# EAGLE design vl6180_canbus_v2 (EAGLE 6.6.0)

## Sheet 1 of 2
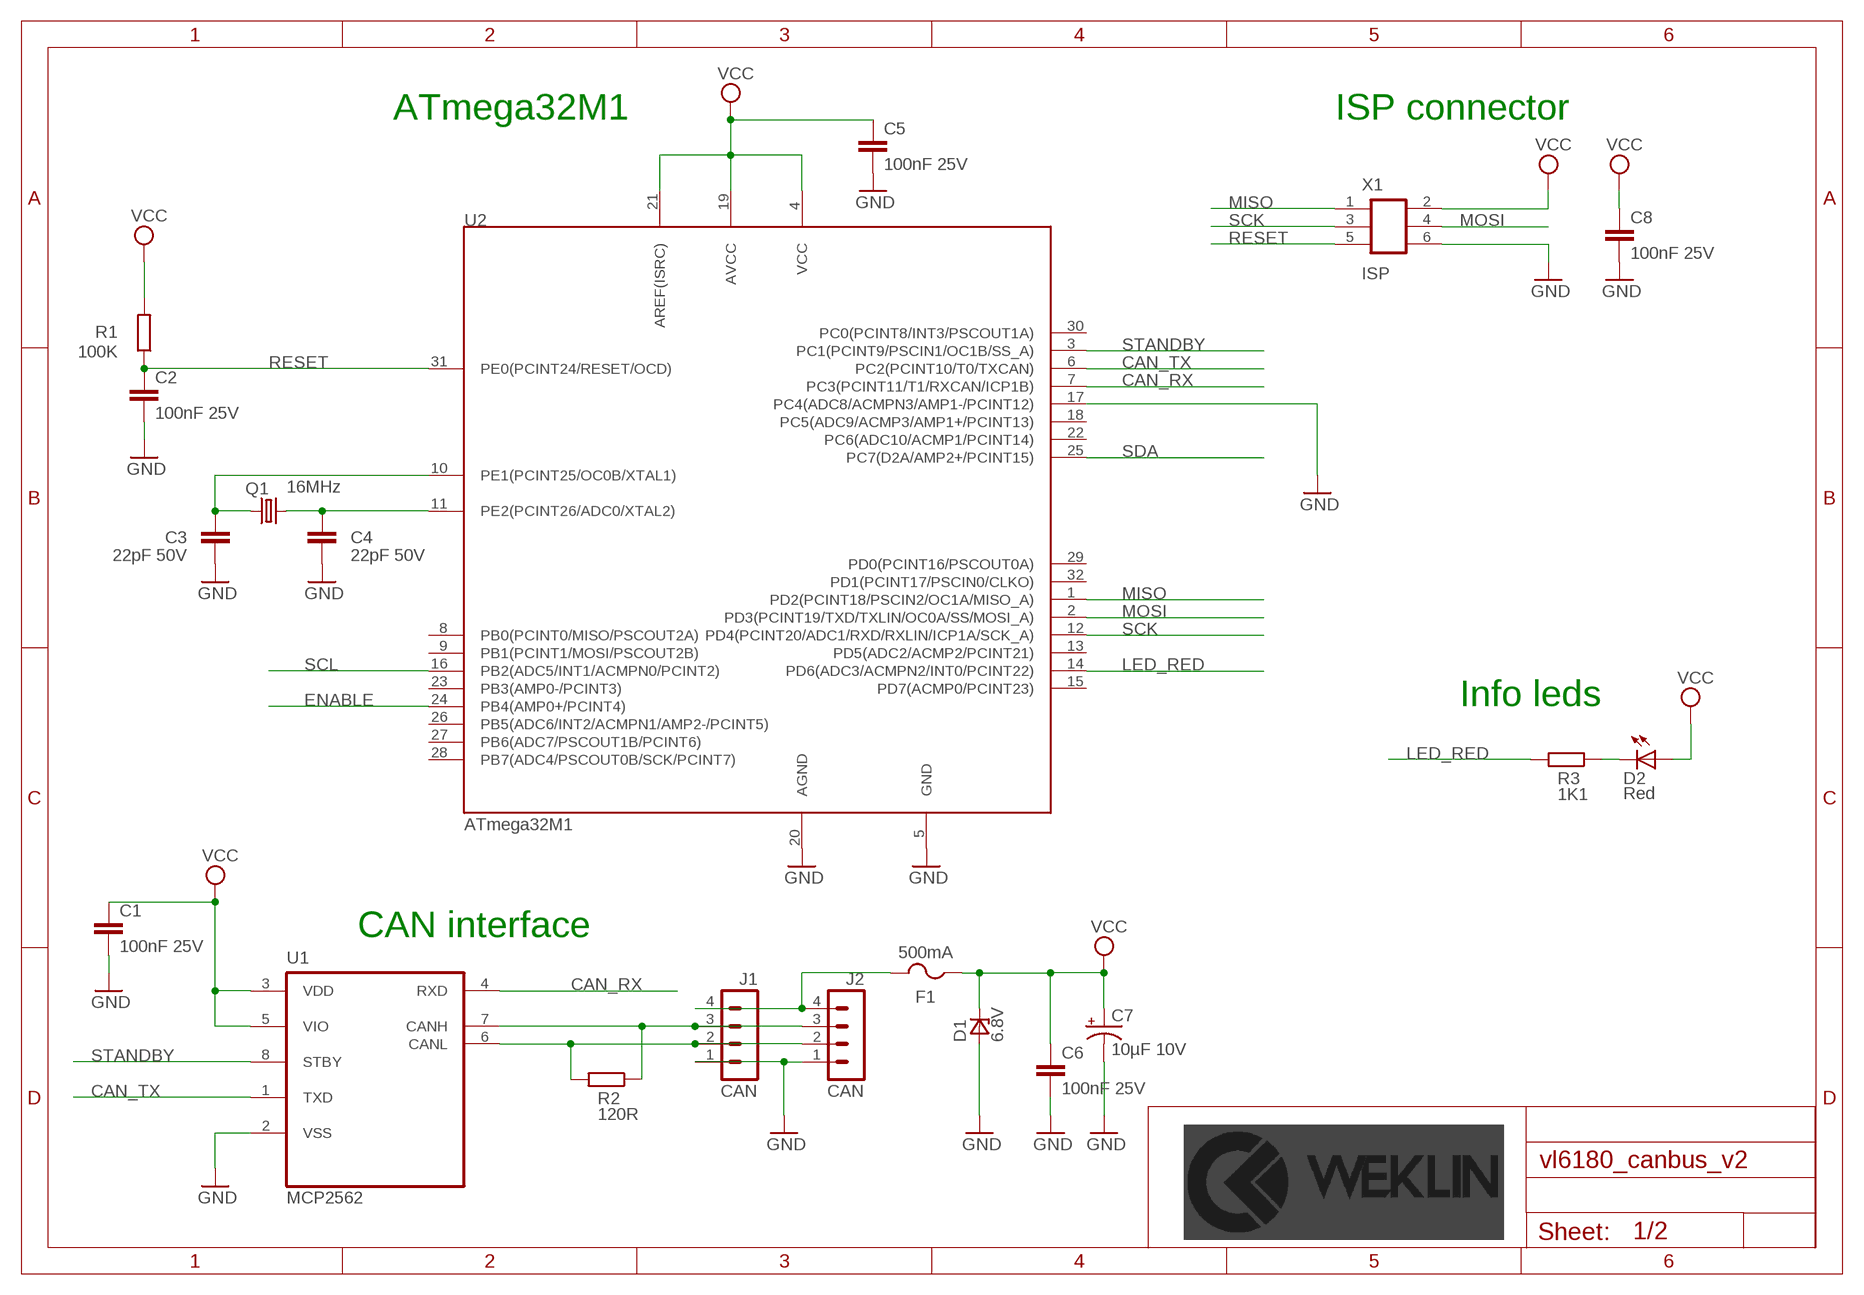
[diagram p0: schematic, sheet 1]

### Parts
C1  100nF 25V  CAPACITOR_NON_POL-100NF-25V(+-10%)(2012)  [C2012]
C2  100nF 25V  CAPACITOR_NON_POL-100NF-25V(+-10%)(2012)  [C2012]
C3  22pF 50V  CAPACITOR_NON_POL-22PF-50V(+-5%)(2012)  [C2012]
C4  22pF 50V  CAPACITOR_NON_POL-22PF-50V(+-5%)(2012)  [C2012]
C5  100nF 25V  CAPACITOR_NON_POL-100NF-25V(+-10%)(2012)  [C2012]
C6  100nF 25V  CAPACITOR_NON_POL-100NF-25V(+-10%)(2012)  [C2012]
C7  10µF 10V  CAPACITOR_POL-10µF-10V(+-10%)(3216)  [EIA3216]
C8  100nF 25V  CAPACITOR_NON_POL-100NF-25V(+-10%)(2012)  [C2012]
D1  6.8V  ZENER_UNIDIR6.8  [DO-214AA]
D2  Red  LEDVLDS1235G  [VLD]
F1  500mA  FUSE0451.500MRL  [EIARS-481-2]
J1  CAN  MICROLOCK-4CMS_VERTICAL  [504194-0470]
J2  CAN  MICROLOCK-4CMS_VERTICAL  [504194-0470]
Q1  16MHz  CRYSTAL-16MHZ_SMD(3225)  [SMD_KX7]
R1  100K  RESISTOR-100K(+-1%)(2012)  [R2012]
R2  120R  RESISTOR-120R(+-1%)(2012)  [R2012]
R3  1K1  RESISTOR-1K1(+-1%)(2012)  [R2012]
U1  MCP2562  MCP2562-E/SN-SOIC8  [SOIC8]
U2  ATmega32M1  ATMEGA32M1-TQFP32  [TQFP32]
X1  ISP  CON_2X3-SMD_1.27MM_MALE  [2X3_1.27MM_MALE_SMD]

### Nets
CAN_RX: U1.4(RXD) U2.7(PC3(PCINT11/T1/RXCAN/ICP1B))
CAN_TX: U1.1(TXD) U2.6(PC2(PCINT10/T0/TXCAN))
ENABLE: U2.24(PB4(AMP0+/PCINT4)) ; also sheet 2
GND: C1.2 C2.2 C3.2 C4.2 C5.2 C6.2 C7.C(-) C8.2 D1.A J1.1 J2.1 U1.2(VSS) U2.5(GND) U2.17(PC4(ADC8/ACMPN3/AMP1-/PCINT12)) U2.20(AGND) X1.6 ; also sheet 2
LED_RED: R3.2 U2.14(PD6(ADC3/ACMPN2/INT0/PCINT22))
MISO: U2.1(PD2(PCINT18/PSCIN2/OC1A/MISO_A)) X1.1
MOSI: U2.2(PD3(PCINT19/TXD/TXLIN/OC0A/SS/MOSI_A)) X1.4
N$2: D2.C R3.1
N$4: F1.2 J1.4 J2.4
N$5: J1.2 J2.2 R2.2 U1.6(CANL)
N$6: J1.3 J2.3 R2.1 U1.7(CANH)
N$7: C4.1 Q1.3 U2.11(PE2(PCINT26/ADC0/XTAL2))
N$9: C3.1 Q1.1 U2.10(PE1(PCINT25/OC0B/XTAL1))
RESET: C2.1 R1.1 U2.31(PE0(PCINT24/RESET/OCD)) X1.5
SCK: U2.12(PD4(PCINT20/ADC1/RXD/RXLIN/ICP1A/SCK_A)) X1.3
SCL: U2.16(PB2(ADC5/INT1/ACMPN0/PCINT2)) ; also sheet 2
SDA: U2.25(PC7(D2A/AMP2+/PCINT15)) ; also sheet 2
STANDBY: U1.8(STBY) U2.3(PC1(PCINT9/PSCIN1/OC1B/SS_A))
VCC: C1.1 C5.1 C6.1 C7.A(+) C8.1 D1.C D2.A F1.1 R1.2 U1.3(VDD) U1.5(VIO) U2.4(VCC) U2.19(AVCC) U2.21(AREF(ISRC)) X1.2 ; also sheet 2
Unconnected: U2.8(PB0(PCINT0/MISO/PSCOUT2A)) U2.9(PB1(PCINT1/MOSI/PSCOUT2B)) U2.13(PD5(ADC2/ACMP2/PCINT21)) U2.15(PD7(ACMP0/PCINT23)) U2.18(PC5(ADC9/ACMP3/AMP1+/PCINT13)) U2.22(PC6(ADC10/ACMP1/PCINT14)) U2.23(PB3(AMP0-/PCINT3)) U2.26(PB5(ADC6/INT2/ACMPN1/AMP2-/PCINT5)) U2.27(PB6(ADC7/PSCOUT1B/PCINT6)) U2.28(PB7(ADC4/PSCOUT0B/SCK/PCINT7)) U2.29(PD0(PCINT16/PSCOUT0A)) U2.30(PC0(PCINT8/INT3/PSCOUT1A)) U2.32(PD1(PCINT17/PSCIN0/CLKO))

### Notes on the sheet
- ATmega32M1 | ISP connector
- Info leds
- CAN interface

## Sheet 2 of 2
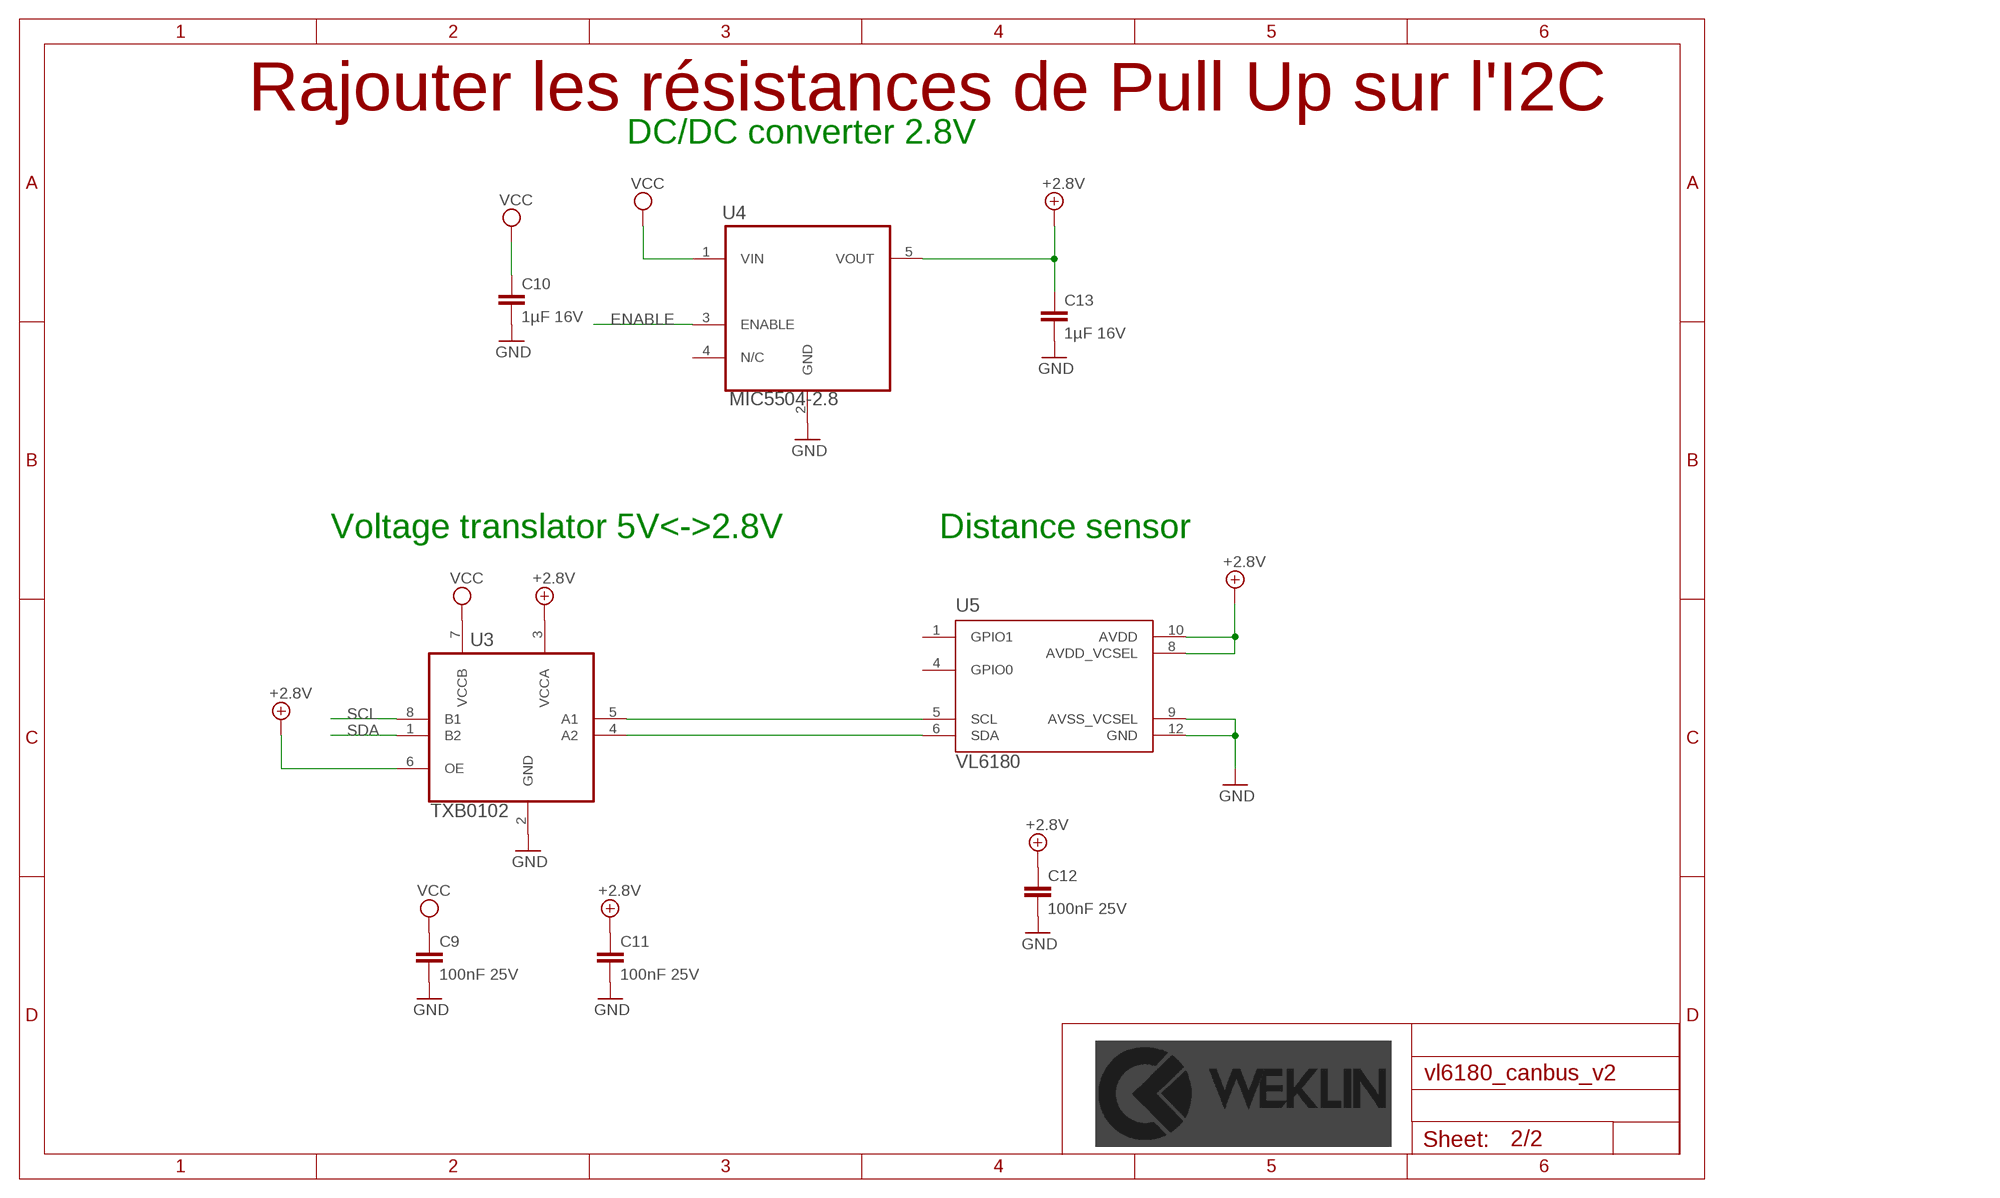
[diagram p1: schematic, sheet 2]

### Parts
C9  100nF 25V  CAPACITOR_NON_POL-100NF-25V(+-10%)(2012)  [C2012]
C10  1µF 16V  CAPACITOR_NON_POL-1µF-16V(-20%)(2012)  [C2012]
C11  100nF 25V  CAPACITOR_NON_POL-100NF-25V(+-10%)(2012)  [C2012]
C12  100nF 25V  CAPACITOR_NON_POL-100NF-25V(+-10%)(2012)  [C2012]
C13  1µF 16V  CAPACITOR_NON_POL-1µF-16V(-20%)(2012)  [C2012]
U3  TXB0102  [VSSOP-8]
U4  MIC5504-2.8  MIC5504-2.8M5-TR  [SOT23-5]
U5  VL6180  [VL6180]

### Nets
+2.8V: C11.1 C12.1 C13.1 U3.3(VCCA) U3.6(OE) U4.5(VOUT) U5.8(AVDD_VCSEL) U5.10(AVDD)
ENABLE: U4.3(ENABLE) ; also sheet 1
GND: C9.2 C10.2 C11.2 C12.2 C13.2 U3.2(GND) U4.2(GND) U5.9(AVSS_VCSEL) U5.12(GND) ; also sheet 1
N$8: U3.5(A1) U5.5(SCL)
N$10: U3.4(A2) U5.6(SDA)
SCL: U3.8(B1) ; also sheet 1
SDA: U3.1(B2) ; also sheet 1
VCC: C9.1 C10.1 U3.7(VCCB) U4.1(VIN) ; also sheet 1
Unconnected: U4.4(N/C) U5.1(GPIO1) U5.4(GPIO0)

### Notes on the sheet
- Rajouter les résistances de Pull Up sur l'I2C
- DC/DC converter 2.8V
- Voltage translator 5V<->2.8V | Distance sensor

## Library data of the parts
C1 C2 C5 C6 C8 C9 C11 C12 = weklin_capacitor:CAPACITOR_NON_POL: Condensateur céramique multicouche; LIB: weklin_capacitor; MANUFACTURER: AVX; MPN: 08053C104KAT2A; OC_FARNELL: 2280951; PRICE: 0,0036
C3 C4 = weklin_capacitor:CAPACITOR_NON_POL: Condensateur céramique multicouche; LIB: weklin_capacitor; MANUFACTURER: Multicomp; MPN: MC0805N220J500CT; OC_FARNELL: 2310684; PRICE: 0,0078
C7 = weklin_capacitor:CAPACITOR_POL: Capacitor; LIB: weklin_capacitor; MANUFACTURER: Kemet; MPN: T491A106K010AT; OC_FARNELL: 2250086; PRICE: 0,0578
C10 C13 = weklin_capacitor:CAPACITOR_NON_POL: Condensateur céramique multicouche; LIB: weklin_capacitor; MANUFACTURER: Walsin; MPN: 0805F105Z160CT; OC_FARNELL: 2495495; PRICE: 0,0097
D1 = weklin_diode:ZENER_UNIDIR: P6SMBxxA Series of unidirectional Transient Voltage Suppressor Diodes; LIB: weklin_diode; MANUFACTURER: ON Semiconductor; MPN: P6SMB6.8AT3G; OC_FARNELL: 1459166RL; PRICE: 0,178
D2 = weklin_led:LED: Led; LIB: weklin_led; MANUFACTURER: Vishay; MPN: VLDS1235G; OC_FARNELL: 2494682; PRICE: 0,003
F1 = weklin_fuse:FUSE: Fuse; LIB: weklin_fuse; MANUFACTURER: Littlefuse; MPN: 0451500MRL; OC_FARNELL: 2383271; PRICE: 0,527
J1 J2 = weklin_micro-lock:MICROLOCK-4: Connecteur MOLEX de 4 Contacts Série Mini50 GEII/IUT ANGERS; LIB: weklin_micro-lock; MANUFACTURER: Molex; MPN: 504194-0470; OC_FARNELL: 2445424; PRICE: 0,232
Q1 = weklin_crystal:CRYSTAL: Crystal resonator; LIB: weklin_crystal; MANUFACTURER: AEL CRYSTALS; MPN: E3SB16.0000F09G11AE; OC_FARNELL: 2467444RL; PRICE: 0,315
R1 = weklin_resistor:RESISTOR: Resistor; LIB: weklin_resistor; MANUFACTURER: Multicomp; MPN: MCWR08X1003FTL; OC_FARNELL: 2446868; PRICE: 0,0014
R2 = weklin_resistor:RESISTOR: Resistor; LIB: weklin_resistor; MANUFACTURER: Multicomp; MPN: MCWR08X1200FTL; OC_FARNELL: 2446878; PRICE: 0,0014
R3 = weklin_resistor:RESISTOR: Resistor; LIB: weklin_resistor; MANUFACTURER: Multicomp; MPN: MC0805S8F1101T5E; OC_FARNELL: 1635316; PRICE: 0,003
U1 = weklin_ic_can:MCP2562-E/SN: High-Speed CAN Transceiver; LIB: weklin_ic_can; MANUFACTURER: Microchip; MPN: MCP2562-E/SN; OC_FARNELL: 2362839; PRICE: 1,12
U2 = weklin_micro-atmell:ATMEGA32M1: ATMEL ATMEGA32M1-AU MCU 8 BITS ATMEGA 16MHZ; LIB: weklin_micro_atmell; MANUFACTURER: Atmel; MPN: ATmega32M1-AU; OC_FARNELL: 2443180; PRICE: 6,18
U3 = weklin_ic_special:TXB0102: Convertisseur de niveau de tension de 1,2V à 5,5V Doc constructeur GEII/IUT ANGERS; LIB: weklin_ic_special; MANUFACTURER: Texas Instrument; MPN: TXB0102DCUR; OC_FARNELL: 2295723; PRICE: 0,962
U4 = weklin_regulator:MIC5504: MICROCHIP MIC5504-2.8YM5-TR Régulateur LDO Tension fixe, 2.5V à 5.5V, 160mV Dropout, 2.8Vout, 300mA, SOT-23-5; LIB: weklin_regulator; MANUFACTURER: Micrel; MNP: MIC5504-2.8YM5-TR; OC_FARNELL: 2510373RL; PRICE: 0.0775
U5 = weklin_sensor:VL6180: Time of flight distance sensor; LIB: weklin_sensor; MANUFACTURER: ST Microelectronics; MPN: VL6180XV0NR/1; OC_FARNELL: 2462820; PRICE: 7,79
X1 = weklin_connector:CON_2X3: Board-To-Board Connector, Micro-MaTch Series, Embase, 6voies.; LIB: weklin_connector; MANUFACTURER: Minitek; MPN: 20021121-00006C4LF; OC_FARNELL: 1865277; PRICE: 0,333

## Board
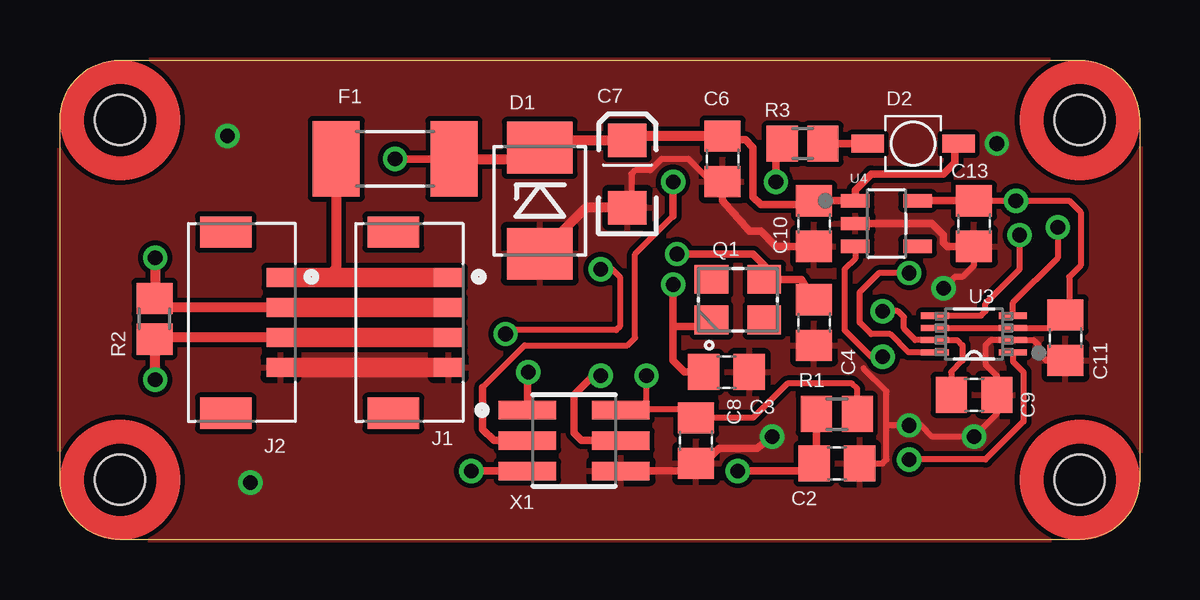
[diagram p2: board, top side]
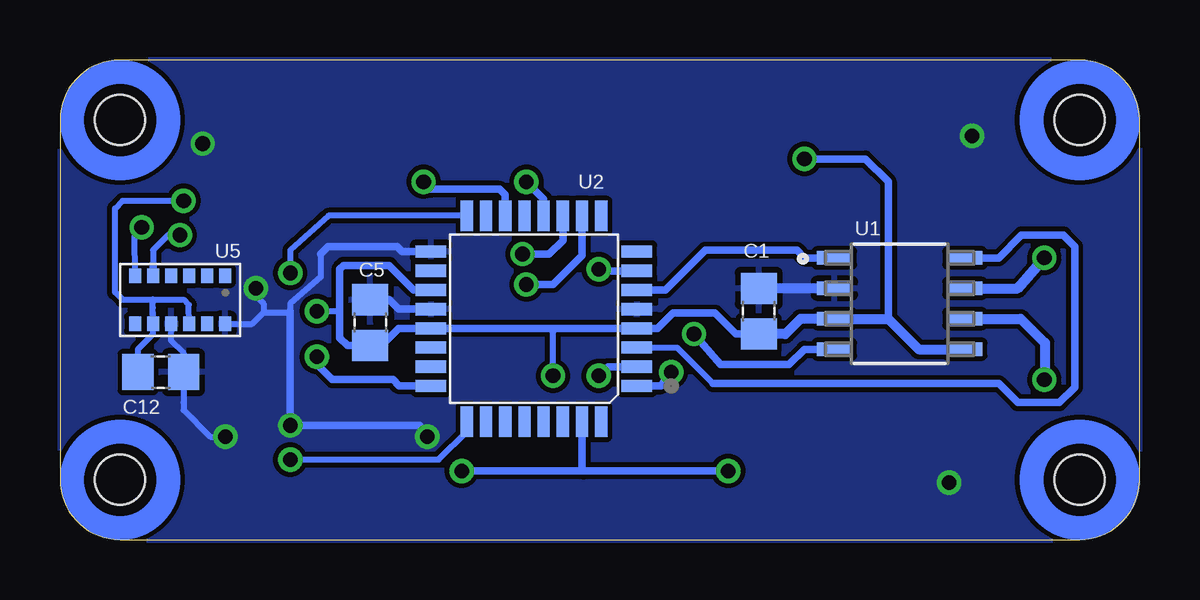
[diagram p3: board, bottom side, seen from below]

Size 45 x 20 mm. Coordinates in mm from the lower left corner, seen from the top.
Outline: 0,2.5 0,17.5 arc-90 2.5,20 42.5,20 arc-90 45,17.5 45,2.5 arc-90 42.5,0 2.5,0 arc-90 0,2.5
Copper layers (1*16): Top 0.035mm / dielectric 1.5mm / Bottom 0.035mm
Design rules "default *": minimum track width 10mil, minimum drill 24mil, track to track 8mil, track to pad 8mil, pad to pad 8mil, via to via 8mil, smd to smd 8mil, copper to edge 0mil, drill to drill 8mil, minimum pad ring 10mil, minimum via ring 8mil, stop-mask expansion 4mil, vias tented up to drill 0mil, thermal gap 10mil
Holes 2.1 mm at 2.5,17.5 42.5,17.5 42.5,2.5 2.5,2.5
tKeepout: area -0.5,14.5 to 5.5,20.5; area -0.5,-0.5 to 5.5,5.5; area 39.5,14.5 to 45.5,20.5; area 39.5,-0.5 to 45.5,5.5; area 2,0 to 42.5,2; area 0,3 to 2,17; area 3,18 to 42.5,20; area 43,3.5 to 45,17
bKeepout: area 3,18 to 42.5,20; area 0,3 to 2,17; area 2,0 to 42.5,2; area 43,3.5 to 45,17; area 39.5,14.5 to 45.5,20.5; area -0.5,14.5 to 5.5,20.5; area -0.5,-0.5 to 5.5,5.5; area 39.5,-0.5 to 45.5,5.5

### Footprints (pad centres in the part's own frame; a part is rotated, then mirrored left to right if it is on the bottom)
C2012 = smd 1.3 x 1.5: 1 -0.95,0; 2 0.95,0
EIA3216 = smd 1.4 x 1.6: A 1.4,0; C -1.4,0
DO-214AA = smd 2.159 x 2.743: A 2.21,0; C -2.21,0
VLD = smd 1.35 x 0.75: A 1.9,0; C -1.9,0
EIARS-481-2 = smd 1.956 x 3.15: 1 -2.451,0; 2 2.451,0
504194-0470 = smd 0.8 x 1.2: 1 -1.875,0; 2 -0.625,0; 3 0.625,0; 4 1.875,0 | smd 1.3 x 2.15: P$5 -3.775,2.295; P$6 3.775,2.295
SMD_KX7 = smd 1.4 x 1.2: 1 -1.1,-0.85; 2 1.1,-0.85; 3 1.1,0.85; 4 -1.1,0.85
R2012 = smd 1.3 x 1.5: 1 -0.85,0; 2 0.85,0
SOIC8 = smd 1.473 x 0.559: 1 -2.718,1.905; 2 -2.718,0.635; 3 -2.718,-0.635; 4 -2.718,-1.905; 5 2.718,-1.905; 6 2.718,-0.635; 7 2.718,0.635; 8 2.718,1.905
TQFP32 = smd 1.27 x 0.508: 1 -4.293,2.8; 2 -4.293,2; 3 -4.293,1.2; 4 -4.293,0.4; 5 -4.293,-0.4; 6 -4.293,-1.2; 7 -4.293,-2; 8 -4.293,-2.8; 17 4.293,-2.8; 18 4.293,-2; 19 4.293,-1.2; 20 4.293,-0.4; 21 4.293,0.4; 22 4.293,1.2; 23 4.293,2; 24 4.293,2.8 | smd 0.508 x 1.27: 9 -2.8,-4.293; 10 -2,-4.293; 11 -1.2,-4.293; 12 -0.4,-4.293; 13 0.4,-4.293; 14 1.2,-4.293; 15 2,-4.293; 16 2.8,-4.293; 25 2.8,4.293; 26 2,4.293; 27 1.2,4.293; 28 0.4,4.293; 29 -0.4,4.293; 30 -1.2,4.293; 31 -2,4.293; 32 -2.8,4.293
VSSOP-8 = smd 1.168 x 0.254: 1 -1.626,0.762; 2 -1.626,0.254; 3 -1.626,-0.254; 4 -1.626,-0.762; 5 1.626,-0.762; 6 1.626,-0.254; 7 1.626,0.254; 8 1.626,0.762
SOT23-5 = smd 0.55 x 1.2: 1 -0.95,-1.3; 2 0,-1.3; 3 0.95,-1.3; 4 0.95,1.3; 5 -0.95,1.3
VL6180 = smd 0.5 x 0.6: 1 -1.875,-1; 2 -1.125,-1; 3 -0.375,-1; 4 0.375,-1; 5 1.125,-1; 6 1.875,-1; 7 1.875,1; 8 1.125,1; 9 0.375,1; 10 -0.375,1; 11 -1.125,1; 12 -1.875,1
2X3_1.27MM_MALE_SMD = smd 2.4 x 0.76: 1 -1.95,1.27; 2 1.95,1.27; 3 -1.95,0; 4 1.95,0; 5 -1.95,-1.27; 6 1.95,-1.27

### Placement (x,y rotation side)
C1  15.88,9.53 90 bottom
C2  32.38,3.17 0 top
C3  27.78,6.99 0 top
C4  31.43,9.05 270 top
C5  32.07,9.05 90 bottom
C6  27.62,15.88 270 top
C7  23.65,15.24 90 top
C8  26.51,4.13 270 top
C9  38.1,6.03 0 top
C10  31.43,13.18 270 top
C11  41.91,8.41 270 top
C12  40.8,6.99 0 bottom
C13  38.1,13.18 270 top
D1  20,14.13 270 top
D2  35.56,16.51 0 top
F1  13.97,15.88 180 top
J1  16.19,9.05 90 top
J2  9.21,9.05 90 top
Q1  28.26,10 0 top
R1  32.38,5.24 0 top
R2  3.94,9.21 270 top
R3  30.96,16.51 180 top
U1  10,9.84 0 bottom
U2  25.24,9.21 180 bottom
U3  38.1,8.57 180 top
U4  34.45,13.18 270 top
U5  40,10 180 bottom
X1  21.43,4.13 0 top

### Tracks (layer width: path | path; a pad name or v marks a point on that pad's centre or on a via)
+2.8V  (via drill 0.61)
  Top 0.254: C13.1 v39.85,14.13 | v39.85,14.13 42.07,14.13 42.55,13.65 42.55,11.43 42.07,10.95 42.07,9.52 C11.1 41.37,8.83 U3.3 U3.6 | v39.85,14.13
  Top 0.305: U4.5 C13.1
  Bottom 0.254: U5.8 41.13,9.67 41.12,10 | 41.12,10 39.85,10 39.63,9.79 U5.10 | C12.1 41.75,7.94 41.13,8.56 U5.8 | U5.8 41.13,10.02 | 41.12,10 42.39,10 42.7,10.32 42.7,13.81 42.39,14.13 v39.85,14.13
CAN_RX  (via drill 0.61)
  Top 0.254: v22.54,11.27 23.02,11.27 23.34,10.95 23.34,8.89 23.18,8.73 18.73,8.73 v18.57,8.57
  Bottom 0.305: v18.57,8.57 17.46,7.3 14.61,7.3 13.97,7.94 U1.4 | U2.7 22.48,11.21 v22.54,11.27
CAN_TX
  Bottom 0.305: U1.1 13.97,11.75 14.29,12.06 18.1,12.06 19.75,10.41 U2.6
ENABLE  (via drill 0.61)
  Top 0.254: U4.3 33.15,11.72 32.7,11.27 32.7,8.73 33.81,7.62 v34.29,7.62
  Bottom 0.305: v34.29,7.62 34.29,7.3 33.66,6.67 31.11,6.67 30.86,6.41 U2.24
GND  (via drill 0.61)
  Top 0.254: 27.14,14.93 26.19,15.88 25.08,15.88 24.61,15.4 23.97,15.4 23.81,15.24 23.81,14 | C2.2 34.29,3.17 34.45,3.33 34.45,4.76 | 34.45,4.76 34.45,6.19 33.5,7.14 | C11.2 41.12,7.46 40.8,7.78 40.8,8.1 40.58,8.32 U3.2 38.8,8.32 38.58,8.1 38.58,7.3 39.05,6.83 C9.2 39.05,5.24 v38.1,4.29 36.35,4.29 35.88,4.76 v35.4,4.76 34.45,4.76 | v36.83,10.48 37.31,10.95 37.62,10.95 38.1,11.43 C13.2 37.62,12.23 37.62,12.22
  Top 0.305: J1.1 14.63,7.17 | C4.2 31.43,7.94 | 27.14,14.93 C6.2 27.62,14.13 28.73,12.86 29.21,12.86 29.84,12.23 C10.2 | 23.81,14 C7.C | X1.6 26.19,2.86 C8.2 26.83,3.18 27.46,3.81 29.05,3.81 v29.69,4.29 | U4.2 36.35,13.18 36.83,12.7 36.83,12.38 36.99,12.22 37.62,12.22 | C11.2
  Top 0.406: C7.C 21.92,13.84 D1.A
  Top 0.813: J2.1 J1.1
  Bottom 0.254: v38.1,4.29 38.73,4.29 39.85,5.4 39.85,5.72 C12.2 39.85,7.78 40.38,8.31 U5.9 | 34.13,11.91 34.13,10.95 35.4,9.84 35.4,9.53 35.45,9.48 36.51,9.48 | v36.83,10.48 36.83,10.16 36.51,9.84 36.51,9.48 | U5.12 36.99,9 36.51,9.48
  Bottom 0.305: U2.20 30.88,9.61 31.27,10 C5.2 | v29.69,4.29 30,4.76 v35.4,4.76 35.4,9.53 | 34.13,11.91 33.81,12.22 30.96,12.22 30.74,12.01 U2.17
  Bottom 0.406: U1.2 C1.2
  other vias: 6.99,16.83 7.94,2.38 39.05,16.51
  pour Top: 2.5,20 42.5,20 arc-90 45,17.5 45,2.5 arc-90 42.5,0 2.5,0 arc-90 0,2.5 0,17.5 arc-90
  pour Bottom: 2.5,20 42.5,20 arc-90 45,17.5 45,2.5 arc-90 42.5,0 2.5,0 arc-90 0,2.5 0,17.5 arc-90
LED_RED  (via drill 0.61)
  Top 0.305: v29.84,14.92 29.84,16.19 30,16.35 30,16.41 R3.2
  Bottom 0.305: U2.14 26.44,14.38 26.67,14.61 29.53,14.61 v29.84,14.92
MISO  (via drill 0.61)
  Top 0.305: X1.1 19.48,6.94 v19.53,6.99
  Bottom 0.305: U2.1 19.95,6.41 v19.53,6.99
MOSI  (via drill 0.61)
  Top 0.305: X1.4 21.75,4.13 21.43,4.45 21.43,6.03 22.23,6.83 v22.54,6.83
  Bottom 0.305: v22.54,6.83 22.16,7.21 U2.2
N$2
  Top 0.305: R3.1 D2.C
N$4
  Top 0.406: F1.2 11.52,11.33 11.11,10.92
  Top 0.813: J2.4 11.11,10.92 J1.4
N$5  (via drill 0.61)
  Top 0.406: J2.2 4.17,8.42 R2.2 3.97,8.18 v3.97,6.67
  Top 0.813: J1.2 J2.2
  Bottom 0.406: U1.6 4.95,9.21 3.94,8.2 3.94,6.53 v3.97,6.67
N$6  (via drill 0.61)
  Top 0.406: J2.3 4.17,9.67 R2.1 3.97,9.92 v3.97,11.75
  Top 0.813: J1.3 J2.3
  Bottom 0.406: U1.7 5.08,10.48 v3.97,11.75
N$7  (via drill 0.61)
  Top 0.305: v25.72,11.91 28.89,11.91 29.37,11.43 29.37,11.02 Q1.3 30.9,10.85 C4.1
  Bottom 0.305: U2.11 24.04,12.47 24.61,11.91 v25.72,11.91
N$8  (via drill 0.61)
  Top 0.254: v40.01,12.7 40.01,11.27 38.58,9.84 38.58,9.53 38.39,9.34 U3.5
  Bottom 0.254: v40.01,12.7 40.48,12.7 41.12,12.06 41.12,11.49
  Bottom 0.305: 41.12,11.49 U5.5
N$9  (via drill 0.61)
  Top 0.305: v25.56,10.64 25.56,8.89 | 25.56,8.89 26.62,8.89 Q1.1 | C3.1 26.04,6.99 25.56,7.46 25.56,7.78 25.56,8.73 25.56,8.89
  Bottom 0.305: U2.10 23.24,11.84 24.45,10.64 v25.56,10.64
N$10  (via drill 0.61)
  Top 0.254: v41.59,13.02 41.59,11.75 39.73,9.88 U3.4
  Bottom 0.254: U5.6 41.88,12.67 v41.59,13.02
RESET  (via drill 0.61)
  Top 0.305: X1.5 v17.14,2.86 | v28.26,2.86 31.12,2.86 C2.1 31.54,3.27 R1.1
  Bottom 0.305: v17.14,2.86 23.18,2.86 | 23.18,2.86 v28.26,2.86 | U2.31 23.24,2.92 23.18,2.86
SCK  (via drill 0.61)
  Top 0.254: 25.56,13.49 23.97,11.91 23.97,8.41 23.65,8.1 19.37,8.1 17.62,6.35
  Top 0.305: v25.56,14.92 25.56,13.49 | X1.3 18.1,4.13 17.62,4.6 17.62,6.35
  Bottom 0.305: U2.12 24.84,14.21 v25.56,14.92
SCL  (via drill 0.61)
  Top 0.254: v35.4,11.11 34.13,11.11 33.34,10.32 33.34,9.05 33.81,8.57 34.61,8.57 35.37,7.81 U3.8
  Bottom 0.254: U2.16 33.81,13.5 35.4,12.06 v35.4,11.11
SDA  (via drill 0.61)
  Top 0.254: U3.1 39.73,7.42 40.16,6.99 40.16,4.92 38.58,3.33 v35.4,3.33
  Bottom 0.254: v35.4,3.33 29.21,3.33 28.04,4.5 U2.25
STANDBY
  Bottom 0.254: U2.3 19.28,8.01 17.78,6.51
  Bottom 0.305: 17.78,6.51 5.87,6.51 5.08,5.71 3.33,5.71 2.7,6.35 2.7,12.22 3.17,12.7 4.92,12.7 5.87,11.75 U1.8
VCC  (via drill 0.61)
  Top 0.254: R1.2 33.23,6.29 33.02,6.51 30.32,6.51 28.89,5.08 C8.1 | C9.1 37.15,6.99 37.62,7.46 37.62,8.1 37.4,8.32 U3.7 35.66,8.32 35.18,8.79 35.18,9.27 34.92,9.53 v34.29,9.53 | X1.2 23.38,5.44 24.29,5.44 | v24.45,6.83 24.45,5.6 24.29,5.44 | 24.29,5.44 26.15,5.44 C8.1
  Top 0.305: F1.1 v13.97,15.88 | 26.19,5.4 C8.1 | C6.1 27.78,16.67 28.57,16.67 28.89,16.35 28.89,14.29 29.21,13.97 31.27,13.97 C10.1 U4.1 33.15,14.57 33.81,15.24 36.83,15.24 37.31,15.72 37.31,16.2 D2.A
  Top 0.406: F1.1 19.54,15.88 D1.C 20.3,16.64 C7.A 23.84,16.82 C6.1
  Bottom 0.254: v34.29,9.53 33.34,9.53 | v24.45,6.83 24.45,8.65 24.61,8.81
  Bottom 0.305: U2.19 30.25,10.41 31.27,11.43 33.18,11.43 33.34,11.27 33.34,9.53 33.34,8.41 33.02,8.1 C5.1 31.91,8.26 31.43,8.26 30.88,8.81 U2.21 24.61,8.81 U2.4 20.09,8.81 19.45,9.44 17.7,9.44 16.83,8.57 C1.1 | v13.97,15.88 11.43,15.88 10.48,14.92 10.48,9.21
  Bottom 0.406: C1.1 14.76,8.57 14.13,9.21 U1.3 10.48,9.21 9.21,7.94 U1.5
(copper drawn outside any net)
  shapes: Bottom circle x4, Top circle x4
